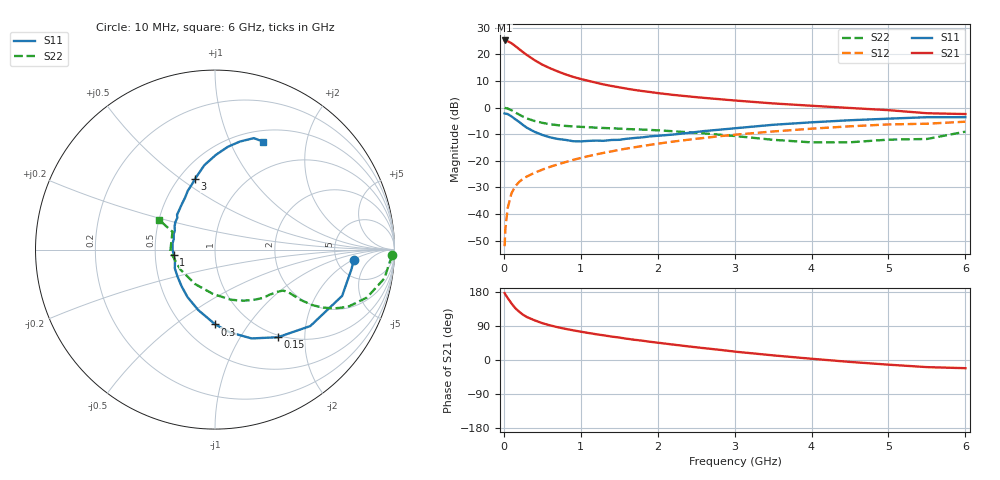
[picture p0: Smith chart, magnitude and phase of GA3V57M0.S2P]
! Infineon Technologies  Discrete & RF Semiconductors
! BF775
! Si NPN RF Bipolar Junction Transistor in SOT23
! VCE = 3.5 V  IC = 7 mA
! Common Emitter S-Parameters:  May  1996
# GHz  S  MA  R  50
!  f  S11  S21  S12  S22
! GHz  MAG  ANG  MAG  ANG  MAG  ANG  MAG  ANG
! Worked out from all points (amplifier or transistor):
!   36 points, 10 MHz to 6 GHz, reference 50 ohm
!   highest |S21| = 25.2 dB at 10 MHz (marker M1)
!   |S21| within 3 dB of that: start of sweep to 188 MHz
!   unconditionally stable (mu >= 1): 687.2 MHz to 3.331 GHz
!   at 250 MHz: K = 0.58, MSG = 23.7 dB, |S12| = -26.7 dB
!   at 1.4 GHz: K = 1.12, MAG = 10.2 dB, |S12| = -16.5 dB
!   at 6 GHz: K = 0.95, MSG = 1.4 dB, |S12| = -5.3 dB
!   S11 on the Smith chart (normalised r, x): 10 MHz: 7.32, -2.09; 150 MHz: 0.97, -1.48; 300 MHz: 0.71, -0.71; 1 GHz: 0.63, -0.04; 3 GHz: 0.60, +0.56; 6 GHz: 0.63, +1.34
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0.01  0.7761 -4.2  18.13 176.6  0.0025 86.8  0.9891 -1.9
0.02  0.7678 -8.3  18.02 173.0  0.0053 88.6  0.9762 -4.0
0.05  0.7538 -20.0  17.52 163.6  0.013 79.5  0.9579 -9.6
0.1  0.6809 -38.7  16.08 149.2  0.0247 72.6  0.8877 -17.5
0.15  0.6006 -54.4  14.18 136.5  0.0334 65.4  0.8065 -23.3
0.2  0.5353 -67.6  12.44 127.3  0.0403 62.2  0.7358 -26.5
0.25  0.4691 -79.7  10.93 119.3  0.0461 60.2  0.6731 -28.5
0.3  0.417 -89.8  9.656 113.3  0.0508 59.7  0.6232 -29.7
0.4  0.3491 -105.6  7.734 104.7  0.0596 58.7  0.5585 -30.4
0.5  0.3057 -120.1  6.372 97.2  0.0682 59.3  0.5156 -30.3
0.6  0.2758 -132.6  5.462 91.4  0.077 60.2  0.4861 -30.2
0.7  0.2572 -144.4  4.761 86.5  0.0855 60.8  0.4663 -30.4
0.8  0.247 -155.0  4.199 82.2  0.0944 61.0  0.452 -30.7
1  0.2316 -172.8  3.434 74.7  0.1131 61.2  0.4338 -32.1
1.1  0.2364 -179.9  3.164 71.3  0.1224 60.9  0.4262 -33.2
1.6  0.2597 150.0  2.254 56.1  0.17 58.8  0.3946 -39.5
2.2  0.3109 127.0  1.726 40.7  0.2293 54.0  0.3589 -50.7
3  0.4075 106.1  1.355 22.2  0.3085 45.5  0.2923 -72.5
3.5  0.4741 97.2  1.194 12.2  0.3551 39.4  0.2478 -92.4
4.5  0.5771 82.9  0.98 -5.1  0.4442 26.3  0.2226 -150.1
5.5  0.6576 70.8  0.781 -18.8  0.4965 11.5  0.2566 157.3
6  0.6588 65.8  0.754 -21.6  0.5421 7.4  0.3523 152.0
